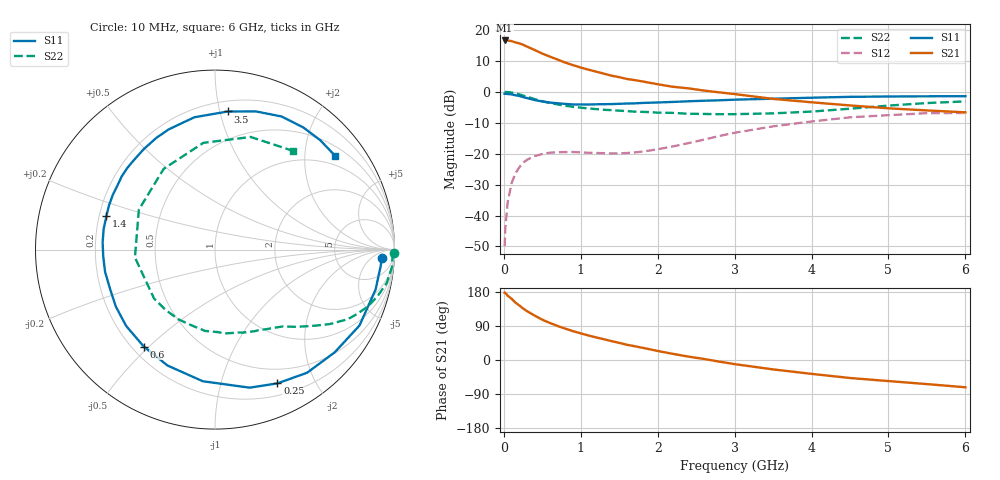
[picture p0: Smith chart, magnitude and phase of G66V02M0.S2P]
! SIEMENS Small Signal Semiconductors
! BFG193
! Si NPN RF Bipolar Junction Transistor in SOT223
! VCE = 6 V  IC = 2 mA
! Common Emitter S-Parameters:  August  1996
# GHz  S  MA  R  50
!  f  S11  S21  S12  S22
! GHz  MAG  ANG  MAG  ANG  MAG  ANG  MAG  ANG
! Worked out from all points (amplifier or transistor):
!   36 points, 10 MHz to 6 GHz, reference 50 ohm
!   highest |S21| = 16.6 dB at 10 MHz (marker M1)
!   |S21| within 3 dB of that: start of sweep to 393.3 MHz
!   unconditionally stable (mu >= 1): 1.368 GHz to 2.512 GHz
!   at 250 MHz: K = 0.17, MSG = 19.1 dB, |S12| = -23.0 dB
!   at 1.4 GHz: K = 1.03, MAG = 11.5 dB, |S12| = -19.9 dB
!   at 6 GHz: K = 0.94, MSG = 0.1 dB, |S12| = -6.8 dB
!   S11 on the Smith chart (normalised r, x): 10 MHz: 19, -13; 250 MHz: 0.33, -1.52; 600 MHz: 0.25, -0.48; 1.4 GHz: 0.23, +0.14; 3.5 GHz: 0.28, +1.06; 6 GHz: 0.73, +2.72
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0.01  0.9299 -2.9  6.76 177.8  0.0032 91.9  0.9951 -1.1
0.02  0.9277 -5.6  6.744 176.9  0.0064 87.5  0.9894 -2.2
0.05  0.922 -14.0  6.73 169.6  0.0164 81.1  0.9909 -5.6
0.1  0.9094 -27.7  6.603 161.7  0.0332 75.2  0.9751 -11.0
0.15  0.8789 -40.6  6.287 151.6  0.0475 67.1  0.942 -16.0
0.2  0.8568 -53.2  6.066 144.1  0.0601 61.0  0.9096 -20.3
0.25  0.8224 -65.0  5.761 136.0  0.071 54.9  0.8688 -24.4
0.3  0.7932 -75.9  5.392 129.0  0.0795 49.8  0.8349 -27.7
0.4  0.7366 -95.3  4.745 117.3  0.0914 40.9  0.762 -33.0
0.5  0.6979 -112.3  4.146 106.3  0.0988 34.0  0.7037 -37.0
0.6  0.6701 -126.3  3.702 97.6  0.1039 29.2  0.6596 -40.4
0.7  0.6527 -139.3  3.311 89.7  0.1055 25.7  0.6251 -43.5
0.8  0.6373 -150.1  2.96 82.6  0.1062 22.5  0.5948 -46.2
1.1  0.624 -176.6  2.277 64.7  0.1036 19.2  0.5376 -54.7
1.4  0.6331 162.9  1.82 49.8  0.1006 20.5  0.5053 -64.1
1.6  0.6462 151.6  1.612 40.2  0.1026 24.2  0.4879 -71.4
2.2  0.6864 125.3  1.206 16.1  0.1313 34.4  0.4563 -97.0
2.8  0.7288 104.5  0.98 -4.3  0.193 32.9  0.4345 -129.5
3.5  0.7728 84.7  0.768 -24.8  0.2764 18.9  0.4483 -174.4
4.5  0.8293 63.4  0.602 -47.5  0.3869 -5.7  0.5332 122.4
5.5  0.8457 46.1  0.5 -63.6  0.4515 -35.0  0.6583 72.4
6  0.849 38.1  0.466 -72.0  0.4546 -50.8  0.7001 51.9
